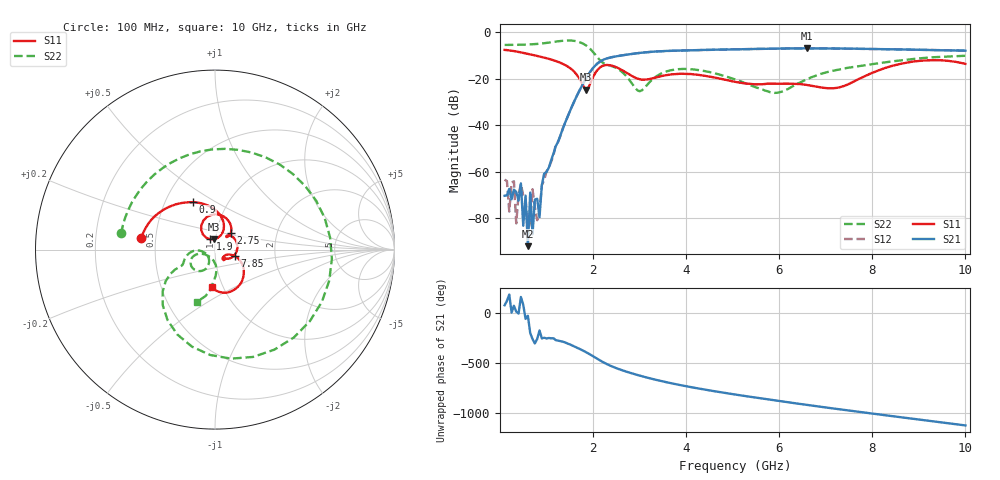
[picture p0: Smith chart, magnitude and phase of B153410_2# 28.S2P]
!  2-Port S-parameters saved by WinCal
! VAR MeasName=S-Parameters (CALIBRATED_DATA) read from VNA (N5245A)
! VAR MeasDate=2016-12-23 10:00:46
! VAR NAME=B153410_2# 28
! VAR FILENAME=B153410_2# 28.S2P
! VAR DATE=2016-12-23 10:00:46
! VAR PHYS_PORTS=1,2
# Hz S DB R 50
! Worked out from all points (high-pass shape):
!   199 points, 100 MHz to 10 GHz, reference 50 ohm
!   highest |S21| = -6.96 dB at 6.6 GHz (marker M1); lowest = -92.1 dB at 600 MHz (marker M2)
!   |S21| within 3 dB of the highest: 2.629 GHz to end of sweep
!   lowest |S11| = -24.8 dB at 1.85 GHz (marker M3), VSWR 1.12, Z = 49.2 + j5.7 ohm
!   |S11| at or under -10 dB: 749.5 MHz to end of sweep
!   |S22| runs from -26.1 to -3.6 dB; largest |S21 - S12| = 0.0036
!   S11 on the Smith chart (normalised r, x): 100 MHz: 0.42, +0.06; 900 MHz: 0.69, +0.40; 1.9 GHz: 0.94, +0.11; 2.75 GHz: 1.17, +0.22; 7.85 GHz: 1.24, -0.09; 10 GHz: 0.89, -0.38
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1e8  -7.64 171.3  -70.43 71.8  -63.48 133.0  -5.51 170.3
2e8  -7.85 162.9  -67.44 178.5  -77.21 -68.7  -5.50 160.4
3e8  -8.14 155.0  -67.78 66.9  -64.19 -56.8  -5.47 150.3
3.5e8  -8.31 151.2  -68.79 8.8  -82.31 -94.5  -5.47 145.0
4.5e8  -8.71 144.0  -65.09 154.4  -65.34 75.4  -5.42 134.4
6e8  -9.34 133.9  -92.13 -32.4  -85.80 -145.5  -5.31 117.2
6.5e8  -9.55 130.7  -69.03 155.9  -81.69 132.0  -5.26 111.1
7e8  -9.78 127.6  -87.03 95.7  -67.65 70.5  -5.21 104.8
8.5e8  -10.46 118.1  -79.69 -178.3  -77.03 -130.6  -4.98 84.4
9e8  -10.71 115.0  -65.80 102.9  -65.85 141.5  -4.88 77.1
1.35e9  -13.65 85.4  -41.67 70.4  -41.38 71.2  -3.70 -4.4
1.75e9  -21.56 68.5  -23.53 -10.2  -23.51 -10.0  -4.62 -92.7
1.85e9  -24.76 94.3  -19.87 -34.4  -19.89 -34.2  -5.72 -114.0
1.9e9  -23.93 114.9  -18.25 -47.4  -18.26 -47.2  -6.49 -124.0
2.75e9  -17.85 46.5  -9.60 127.2  -9.61 127.3  -19.76 -177.5
3.4e9  -19.25 46.2  -8.27 45.8  -8.28 45.9  -18.52 -115.6
5.05e9  -21.40 -36.6  -7.38 -95.0  -7.39 -94.7  -20.33 -165.7
6.6e9  -22.76 -51.1  -6.96 161.6  -6.97 161.6  -20.22 -86.3
6.7e9  -23.11 -51.3  -6.97 155.2  -6.97 155.3  -19.36 -86.0
7.85e9  -18.81 -17.6  -7.20 84.5  -7.19 84.7  -14.17 -94.3
8.35e9  -14.95 -29.9  -7.36 54.7  -7.35 55.0  -12.77 -97.4
1e10  -13.64 -95.0  -7.97 -42.4  -7.95 -42.3  -10.17 -109.3
